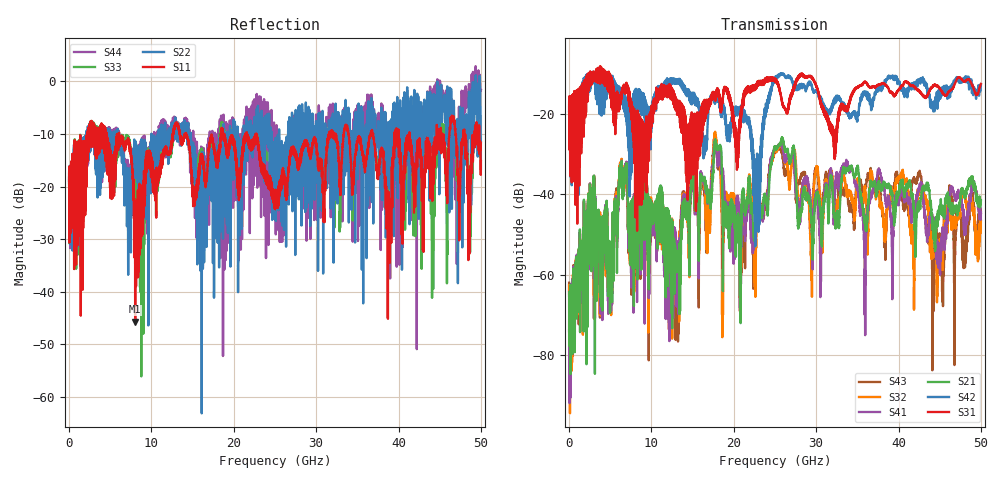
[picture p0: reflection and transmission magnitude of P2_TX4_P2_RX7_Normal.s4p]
!Keysight Technologies,N5225B,MY57041031,A.13.20.10
!Date: Friday, May 31, 2019 11:37:49
!Correction: S11(Full 4 Port(1,2,3,4))
!S12(Full 4 Port(1,2,3,4))
!S13(Full 4 Port(1,2,3,4))
!S14(Full 4 Port(1,2,3,4))
!S21(Full 4 Port(1,2,3,4))
!S22(Full 4 Port(1,2,3,4))
!S23(Full 4 Port(1,2,3,4))
!S24(Full 4 Port(1,2,3,4))
!S31(Full 4 Port(1,2,3,4))
!S32(Full 4 Port(1,2,3,4))
!S33(Full 4 Port(1,2,3,4))
!S34(Full 4 Port(1,2,3,4))
!S41(Full 4 Port(1,2,3,4))
!S42(Full 4 Port(1,2,3,4))
!S43(Full 4 Port(1,2,3,4))
!S44(Full 4 Port(1,2,3,4))
!S4P File: Measurements: <S11,S12,S13,S14>,
!<S21,S22,S23,S24>,
!<S31,S32,S33,S34>,
!<S41,S42,S43,S44>:
# Hz S  dB  R 50.0
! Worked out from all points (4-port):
!   5000 points, 10 MHz to 50 GHz, reference 50 ohm
!   strongest paths, dB at 10 MHz, 12.51 GHz, 25.01 GHz, 37.51 GHz, 50 GHz:
!     S31: -19.3, -14.3, -11.3, -12.8, -12.5
!     S42: -19.4, -12.2, -11.7, -13.8, -12.7
!     S21: -64.3, -50.6, -28.6, -37.1, -41.6
!     S41: -74.2, -52.0, -28.5, -34.0, -44.5
!     S32: -62.7, -50.4, -29.3, -38.1, -46.6
!     S43: -62.1, -52.1, -29.7, -35.6, -44.6
!   lowest |S11| = -45.7 dB at 8.03 GHz (marker M1), VSWR 1.01, Z = 50.3 - j0.455 ohm
!   |S11| at or under -10 dB: 6.073 GHz to 12.61 GHz (6.542 GHz wide, 70 % of centre); 14.21 GHz to 18.43 GHz (4.228 GHz wide, 25.9 % of centre); 22.71 GHz to 31.52 GHz (8.808 GHz wide, 32.5 % of centre)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
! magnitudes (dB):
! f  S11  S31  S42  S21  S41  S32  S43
! 10 MHz  -19.0  -19.3  -19.4  -64.3  -74.2  -62.7  -62.1
! 8.03 GHz  -45.7  -23.4  -14.8  -58.4  -53.2  -49.4  -50.1
! 17.79 GHz  -14.2  -15.3  -16.8  -26.7  -27.2  -25.2  -26.0
! 18.76 GHz  -11.2  -14.1  -18.6  -43.2  -35.9  -46.3  -43.5
! 22.85 GHz  -10.8  -12.1  -36.3  -40.7  -41.1  -41.8  -42.2
! 25.65 GHz  -19.8  -14.7  -10.3  -27.6  -27.8  -27.7  -28.5
! 50 GHz  -15.2  -12.5  -12.7  -41.6  -44.5  -46.6  -44.6
